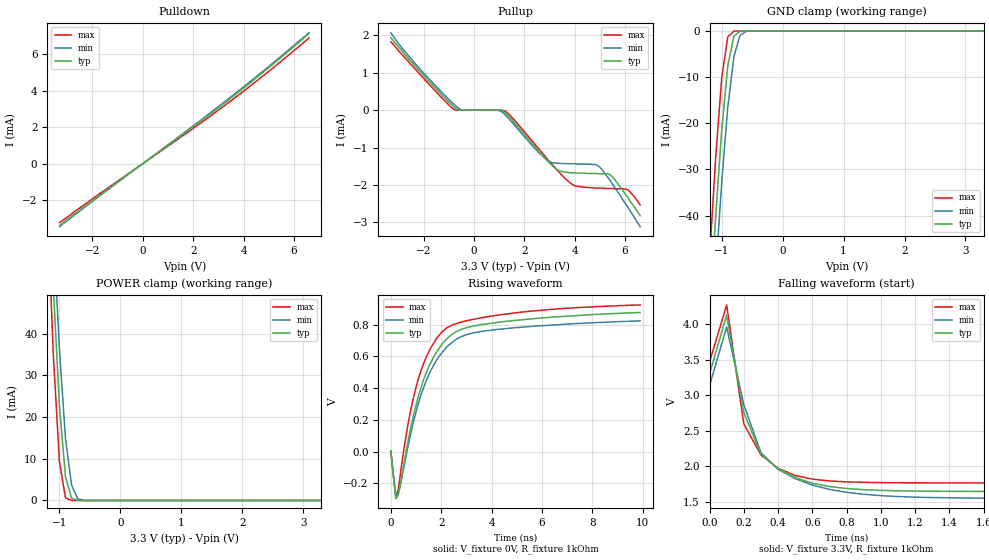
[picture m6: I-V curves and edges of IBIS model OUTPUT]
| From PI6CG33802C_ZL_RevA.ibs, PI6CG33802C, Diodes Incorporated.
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[Model] OUTPUT
Model_type Output
Vmeas =  0.1
Vref = 0
Rref = 1k
| variable   typ   min   max
C_comp   4.138pF   4.098pF   4.182pF
[Voltage Range]   3.3V   3.135V   3.465V
[GND Clamp Reference]   0.000V   0.000V   0.000V
[POWER Clamp Reference]   3.3V   3.135V   3.465V
[Pulldown Reference]   0.000V   0.000V   0.000V
[Pullup Reference]   3.3V   3.135V   3.465V
[temperature range]   25   85   -40
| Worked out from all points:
|   slope of the pulldown table from 0 to 0.495 V, typ, clamps not added: 990 ohm
|   GND clamp passes 1 mA (typ) near -0.79 V on its own axis
|   POWER clamp passes 1 mA (typ) near -0.81 V on its own axis
|   falling waveform, V_fixture 3.3V, R_fixture 1kOhm: 20-80 % time 211ps typ, 265ps min, 161ps max; typ from 3.3 V to 1.64 V
|   rising waveform, V_fixture 0V, R_fixture 1kOhm: 20-80 % time 1.34ns typ, 1.36ns min, 1.25ns max; typ from 0.002 V to 0.877 V
[GND Clamp]
| Voltage   I(typ)   I(min)   I(max)
-3.3V     -611mA     -617mA     -607mA
-1.2V     -62.2mA    -74.3mA    -49.3mA
-1.1V     -40.5mA    -52.6mA    -27.7mA
-1V       -21.5mA    -32.9mA    -10.2mA
-900mV    -7.54mA    -16.5mA    -1.27mA
-800mV    -1.13mA    -5.57mA    -24.2uA
-700mV    -53.2uA    -958uA     -202nA
-600mV    -1.35uA    -74.3uA    -1.53nA
3.3V      9.9pA      35.5pA     9.41pA
[POWER Clamp]   |Note: Vtable = Vcc - Voutput
| Voltage   I(typ)   I(min)   I(max)
-3.3V     1.02A      977mA      1.08A
-1.2V     86.3mA     99mA       71.7mA
-1.1V     51.3mA     65.5mA     35.1mA
-1V       22.8mA     36.4mA     9.39mA
-900mV    5.72mA     14.9mA     638uA
-800mV    544uA      3.68mA     8.25uA
-700mV    18.7uA     441uA      62.5nA
-600mV    428nA      26.6uA     460pA
3.3V      -9.9pA     -97pA      -9.41pA
[Pulldown]
| Voltage   I(typ)   I(min)   I(max)
-3.3V     -3.4mA     -3.46mA    -3.24mA
-1.7V     -1.72mA    -1.76mA    -1.64mA
1.7V      1.72mA     1.76mA     1.64mA
3.2V      3.29mA     3.35mA     3.14mA
5.2V      5.5mA      5.57mA     5.29mA
6.6V      7.15mA     7.19mA     6.91mA
[Pullup]
| Voltage   I(typ)   I(min)   I(max)
-3.3V     1.94mA     2.07mA     1.83mA
-2.3V     1.16mA     1.22mA     1.08mA
-1V       223uA      295uA      142uA
-600mV    7.71uA     50.9uA     2.81uA
1.2V      -44.1uA    -94.8uA    -7.88uA
2.6V      -1.12mA    -1.15mA    -1.05mA
3.3V      -1.59mA    -1.41mA    -1.6mA
4V        -1.67mA    -1.43mA    -2.02mA
5V        -1.7mA     -1.52mA    -2.08mA
5.5V      -1.78mA    -1.97mA    -2.09mA
6.1V      -2.32mA    -2.58mA    -2.12mA
6.6V      -2.82mA    -3.11mA    -2.53mA
[Falling Waveform]
V_fixture = 3.3V
V_fixture_min = 3.135V
V_fixture_max = 3.465V
R_fixture = 1kOhm
C_fixture = 0F
|   Time   V(typ)   V(min)   V(max)
0s        3.3V       3.135V     3.465V
100ps     4.126V     3.96V      4.272V
200ps     2.756V     2.869V     2.596V
300ps     2.169V     2.189V     2.158V
400ps     1.962V     1.955V     1.969V
500ps     1.838V     1.824V     1.868V
700ps     1.713V     1.672V     1.791V
1ns       1.658V     1.584V     1.768V
1.6ns     1.643V     1.549V     1.763V
9.9ns     1.639V     1.541V     1.761V
[Rising Waveform]
V_fixture = 0V
V_fixture_min = 0V
V_fixture_max = 0V
R_fixture = 1kOhm
C_fixture = 0F
|   Time   V(typ)   V(min)   V(max)
0s        2.4mV      2.69mV     186uV
200ps     -297mV     -279mV     -288mV
300ps     -273mV     -260mV     -236mV
700ps     77.5mV     46.1mV     188mV
1.1ns     353mV      306mV      463mV
1.6ns     565mV      515mV      658mV
2.2ns     707mV      655mV      778mV
2.8ns     771mV      726mV      817mV
3.8ns     805mV      763mV      849mV
9.9ns     877mV      825mV      925mV
[Ramp]
|   typ   min   max
dV/dt_r   0.64/1.34E-12   0.62/1.37E-12   0.66/1.23E-12
dV/dt_f   1.49/0.18E-12   1.47/0.22E-12   1.51/0.14E-12
R_load =   1000.0000
